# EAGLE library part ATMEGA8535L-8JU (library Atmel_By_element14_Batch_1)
Microcontroller with 8K Bytes In-System Programmable Flash
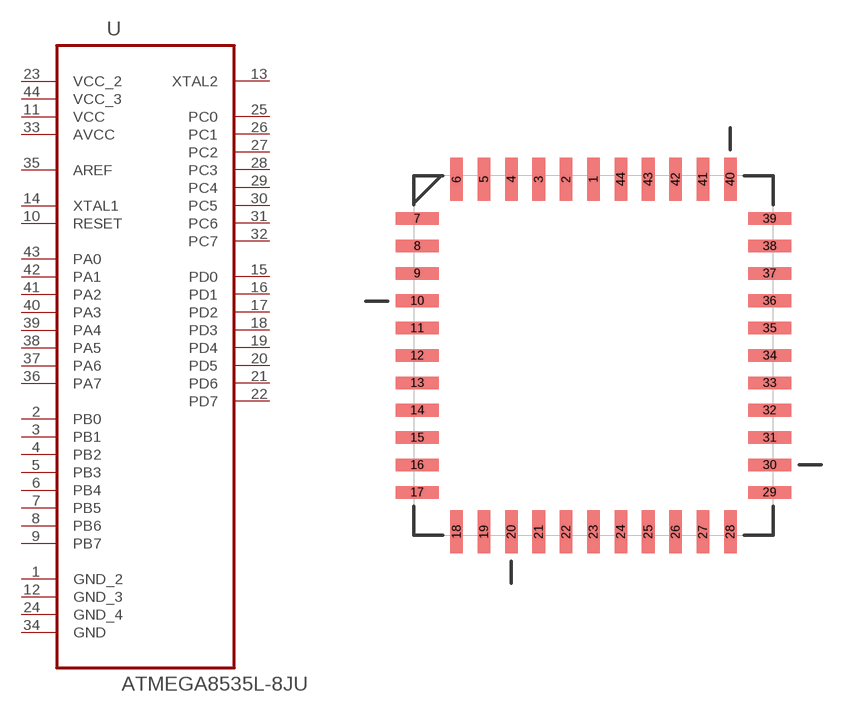
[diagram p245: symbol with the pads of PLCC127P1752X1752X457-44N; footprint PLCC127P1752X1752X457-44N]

Designator prefix U

## ATMEGA8535L-8JU (MPN: ATMEGA8535L-8JU; OC_FARNELL: 1562627; OC_NEWARK: 94M6264; PACKAGE: PLCC-44; SUPPLIER: Atmel)  [PLCC127P1752X1752X457-44N]
1  GND_2  pas
2  PB0
3  PB1
4  PB2
5  PB3
6  PB4
7  PB5
8  PB6
9  PB7
10  RESET  in
11  VCC  pwr
12  GND_3  pas
13  XTAL2  out
14  XTAL1  in
15  PD0
16  PD1
17  PD2
18  PD3
19  PD4
20  PD5
21  PD6
22  PD7
23  VCC_2  pwr
24  GND_4  pas
25  PC0
26  PC1
27  PC2
28  PC3
29  PC4
30  PC5
31  PC6
32  PC7
33  AVCC  pwr
34  GND  pas
35  AREF  in
36  PA7
37  PA6
38  PA5
39  PA4
40  PA3
41  PA2
42  PA1
43  PA0
44  VCC_3  pwr

## Footprint PLCC127P1752X1752X457-44N (pad centres in mm)
smd 0.584 x 2.007: 1 0,8.179; 2 -1.27,8.179; 3 -2.54,8.179; 4 -3.81,8.179; 5 -5.08,8.179; 6 -6.35,8.179; 18 -6.35,-8.179; 19 -5.08,-8.179; 20 -3.81,-8.179; 21 -2.54,-8.179; 22 -1.27,-8.179; 23 0,-8.179; 24 1.27,-8.179; 25 2.54,-8.179; 26 3.81,-8.179; 27 5.08,-8.179; 28 6.35,-8.179; 40 6.35,8.179; 41 5.08,8.179; 42 3.81,8.179; 43 2.54,8.179; 44 1.27,8.179
smd 2.007 x 0.584: 7 -8.179,6.35; 8 -8.179,5.08; 9 -8.179,3.81; 10 -8.179,2.54; 11 -8.179,1.27; 12 -8.179,0; 13 -8.179,-1.27; 14 -8.179,-2.54; 15 -8.179,-3.81; 16 -8.179,-5.08; 17 -8.179,-6.35; 29 8.179,-6.35; 30 8.179,-5.08; 31 8.179,-3.81; 32 8.179,-2.54; 33 8.179,-1.27; 34 8.179,0; 35 8.179,1.27; 36 8.179,2.54; 37 8.179,3.81; 38 8.179,5.08; 39 8.179,6.35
